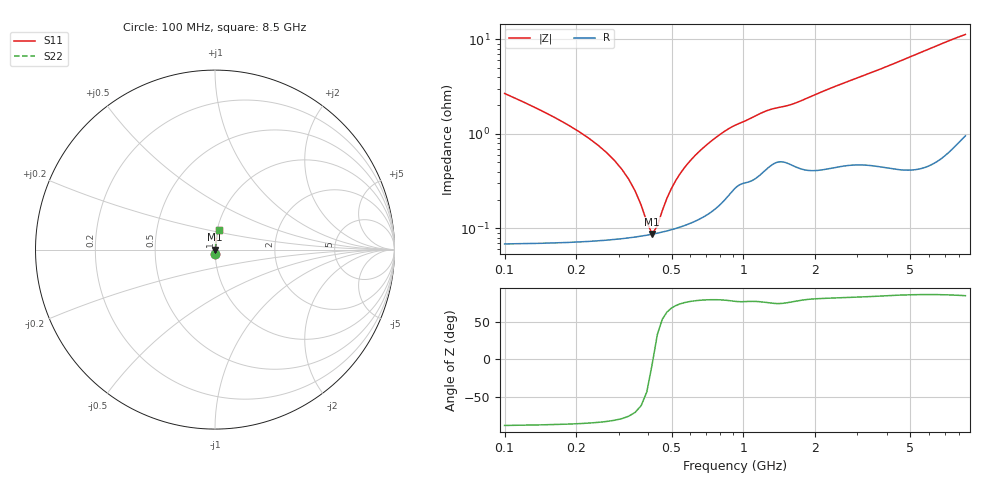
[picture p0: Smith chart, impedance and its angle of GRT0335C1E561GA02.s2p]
!Murata Part Number: GRT0335C1E561GA02
!These Parameters are Measured in Series Mode Connection
!Data Generated on Jun 19, 2026
!  o--ll--o
!Port1  Port2
!  o------o
!Operation Temp=25[degC], DC Bias Voltage=0[V]
!Freq. Start=100[MHz] Stop=9[GHz] 401[Steps]
# Hz S RI R 50
!Freq.(Hz) S11(Real) S11(Imag) S21(Real) S21(Imag) S12(Real) S12(Imag) S22(Real) S22(Imag)
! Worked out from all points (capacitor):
!   401 points, 100 MHz to 8.5 GHz, reference 50 ohm
!   read as one part in series: C = 559 pF near 142 MHz
!   lowest |Z| = 87.3 mohm at 415 MHz (marker M1)
!   series resonance near 418 MHz, so ESL is about 260 pH
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1e8  0.0014 -0.0267  0.9986 0.0267  0.9986 0.0267  0.0014 -0.0267
1.42e8  0.00101 -0.0177  0.999 0.0177  0.999 0.0177  0.00101 -0.0177
2.68e8  0.000789 -0.00625  0.9992 0.00625  0.9992 0.00625  0.000789 -0.00625
3.31e8  0.000803 -0.00321  0.9992 0.00321  0.9992 0.00321  0.000803 -0.00321
3.73e8  0.00083 -0.00156  0.9992 0.00156  0.9992 0.00156  0.00083 -0.00156
3.94e8  0.000847 -0.000806  0.9992 0.000806  0.9992 0.000806  0.000847 -0.000806
4.15e8  0.000867 -9.57e-05  0.9991 9.57e-05  0.9991 9.57e-05  0.000867 -9.57e-05
4.36e8  0.000889 0.00058  0.9991 -0.00058  0.9991 -0.00058  0.000889 0.00058
4.57e8  0.000914 0.00123  0.9991 -0.00123  0.9991 -0.00123  0.000914 0.00123
5.2e8  0.00101 0.00303  0.999 -0.00303  0.999 -0.00303  0.00101 0.00303
5.62e8  0.00108 0.00414  0.9989 -0.00414  0.9989 -0.00414  0.00108 0.00414
6.46e8  0.00127 0.00622  0.9987 -0.00622  0.9987 -0.00622  0.00127 0.00622
7.51e8  0.00163 0.00865  0.9984 -0.00865  0.9984 -0.00865  0.00163 0.00865
8.98e8  0.00261 0.0116  0.9974 -0.0116  0.9974 -0.0116  0.00261 0.0116
1.15e9  0.00375 0.0155  0.9963 -0.0155  0.9963 -0.0155  0.00375 0.0155
1.507e9  0.00529 0.0189  0.9947 -0.0189  0.9947 -0.0189  0.00529 0.0189
2.221e9  0.00504 0.0286  0.995 -0.0286  0.995 -0.0286  0.00504 0.0286
2.914e9  0.00607 0.0374  0.9939 -0.0374  0.9939 -0.0374  0.00607 0.0374
4.3e9  0.00728 0.0552  0.9927 -0.0552  0.9927 -0.0552  0.00728 0.0552
5.707e9  0.00993 0.0742  0.9901 -0.0742  0.9901 -0.0742  0.00993 0.0742
7.114e9  0.0148 0.0929  0.9852 -0.0929  0.9852 -0.0929  0.0148 0.0929
8.5e9  0.0216 0.109  0.9784 -0.109  0.9784 -0.109  0.0216 0.109
